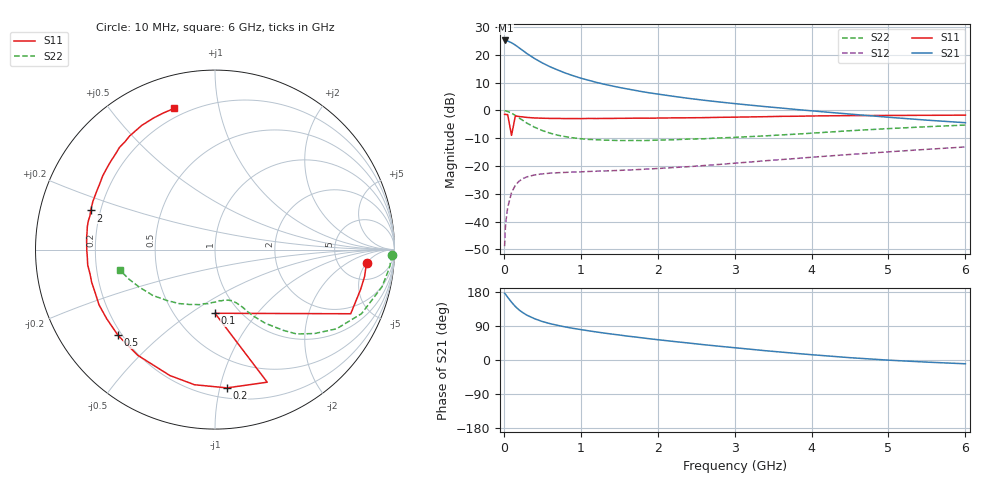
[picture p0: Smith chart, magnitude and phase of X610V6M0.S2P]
! SIEMENS Small Signal Semiconductors
! BFP193W
! Si NPN RF Bipolar Junction Transistor in SOT343
! VCE = 10 V  IC = 6 mA
! Common Emitter S-Parameters:  April 1994
# GHz  S  MA  R  50
!  f  S11  S21  S12  S22
! GHz  MAG  ANG  MAG  ANG  MAG  ANG  MAG  ANG
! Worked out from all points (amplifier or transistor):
!   40 points, 10 MHz to 6 GHz, reference 50 ohm
!   highest |S21| = 25.1 dB at 20 MHz (marker M1)
!   |S21| within 3 dB of that: start of sweep to 215.7 MHz
!   unconditionally stable (mu >= 1): 1.677 GHz to 4.467 GHz
!   at 200 MHz: K = 0.16, MSG = 24.0 dB, |S12| = -25.4 dB
!   at 1.5 GHz: K = 0.94, MSG = 14.9 dB, |S12| = -21.6 dB
!   at 6 GHz: K = 0.92, MSG = 4.4 dB, |S12| = -13.2 dB
!   S11 on the Smith chart (normalised r, x): 10 MHz: 10, -5; 100 MHz: 0.78, -0.63; 200 MHz: 0.27, -1.05; 500 MHz: 0.18, -0.37; 2 GHz: 0.16, +0.15; 6 GHz: 0.15, +0.74
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0.01  0.8476 -4.9  18.04 176.0  0.0036 84.2  0.984 -1.7
0.02  0.8469 -10.2  18.08 174.0  0.0076 80.6  0.979 -5.2
0.05  0.8364 -25.3  17.66 165.6  0.0179 76.4  0.953 -12.6
0.1  0.3548 -90.0  16.44 152.6  0.0331 65.4  0.8912 -23.6
0.15  0.7941 -68.5  14.9 141.0  0.0449 55.9  0.8083 -33.1
0.2  0.7732 -85.1  13.27 131.8  0.0534 48.9  0.7258 -40.1
0.25  0.7615 -98.6  11.83 124.5  0.0595 43.0  0.6549 -45.9
0.3  0.7453 -109.7  10.51 118.3  0.0635 38.7  0.5888 -49.8
0.4  0.7294 -126.2  8.543 108.9  0.0689 32.9  0.4965 -55.7
0.5  0.7213 -138.5  7.132 101.6  0.072 29.4  0.4331 -59.6
0.6  0.7159 -147.4  6.085 96.0  0.0741 27.0  0.3888 -62.4
0.7  0.7157 -154.5  5.324 91.4  0.0754 25.7  0.3571 -64.3
0.9  0.7108 -165.2  4.199 83.5  0.0775 24.8  0.32 -68.1
1.1  0.7144 -173.0  3.481 77.1  0.0795 25.1  0.2999 -71.5
1.3  0.7144 -179.9  2.959 71.2  0.0813 26.0  0.2914 -75.2
1.5  0.7183 174.7  2.584 66.0  0.0831 27.5  0.2864 -79.2
2  0.7264 162.5  1.962 53.6  0.0899 31.9  0.2916 -88.6
2.2  0.7313 158.5  1.791 49.1  0.0933 33.5  0.2953 -93.0
3.2  0.7612 139.7  1.241 28.5  0.1176 39.6  0.3369 -114.7
4.5  0.8034 120.5  0.856 6.1  0.1607 40.1  0.4299 -143.5
5.5  0.8136 110.7  0.666 -5.6  0.1987 37.0  0.5072 -161.1
6  0.8192 106.1  0.599 -10.0  0.2194 35.1  0.5435 -168.1
